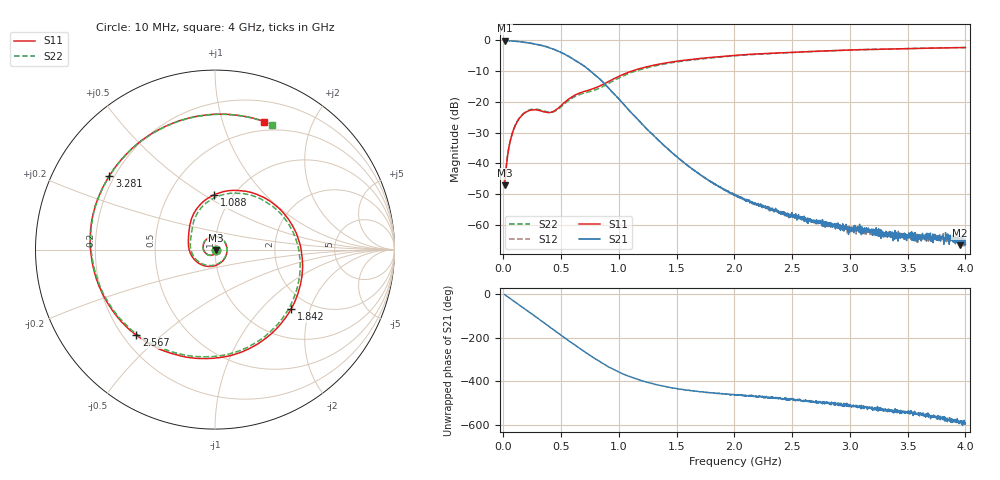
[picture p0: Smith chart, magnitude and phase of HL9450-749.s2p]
! 7/13/2020 7:49:31 AM
! H:\PRODUCTION_DATA\9450\10010\HL9450_10009_467MHZ_.S2P
! CHANNEL.1
! TR.MEASUREMENT
! CORRECTED.DATA
# GHZ S RI R 50.0
! FREQ.GHZ  S11RE  S11IM  S21RE  S21IM  S12RE  S12IM  S22RE  S22IM
!; PortSelection: Port_12
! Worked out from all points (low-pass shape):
!   2000 points, 10 MHz to 4 GHz, reference 50 ohm
!   highest |S21| = -0.04 dB at 10 MHz (marker M1); lowest = -66.7 dB at 3.952 GHz (marker M2)
!   |S21| within 3 dB of the highest: start of sweep to 444.1 MHz
!   lowest |S11| = -47.2 dB at 10 MHz (marker M3), VSWR 1.01, Z = 50.4 - j0.132 ohm
!   |S11| at or under -10 dB: start of sweep to 1.112 GHz
!   |S22| runs from -47.2 to -2.3 dB; largest |S21 - S12| = 0.0036
!   S11 on the Smith chart (normalised r, x): 10 MHz: 1.01, -0.00; 1.088 GHz: 0.82, +0.55; 1.842 GHz: 1.61, -1.50; 2.567 GHz: 0.25, -0.42; 3.281 GHz: 0.18, +0.31; 4 GHz: 0.40, +1.38
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0.01  0.00419 -0.00131  0.9926 -0.068  0.9946 -0.0685  0.00417 -0.00131
0.08185593  -0.0125 -0.0303  0.8355 -0.5062  0.8354 -0.5069  -0.013 -0.0306
0.2036118  -0.0655 0.0229  0.2095 -0.8929  0.2095 -0.8938  -0.0666 0.0239
0.2914357  -0.0112 0.0727  -0.2885 -0.807  -0.2886 -0.8069  -0.0115 0.0746
0.3932316  0.0654 0.0125  -0.6554 -0.3927  -0.656 -0.3929  0.0655 0.0145
0.5449275  -0.0449 -0.0933  -0.5125 0.261  -0.5121 0.2617  -0.0444 -0.0877
0.6766633  -0.1422 -0.00551  -0.1048 0.3926  -0.1036 0.3925  -0.1349 0.00216
0.8383392  -0.1436 0.1127  0.1531 0.1729  0.1519 0.1743  -0.1282 0.1105
1.087839  -0.00595 0.3047  0.0694 -0.021  0.0695 -0.021  3.89e-05 0.2904
1.341331  0.3045 0.2715  0.013 -0.0199  0.0129 -0.0199  0.3009 0.2543
1.586838  0.4792 0.00273  0.00165 -0.0093  0.00168 -0.0092  0.4683 -0.011
1.842326  0.4244 -0.3301  -0.000322 -0.00446  -0.000312 -0.00447  0.4056 -0.3377
2.005998  0.2798 -0.4969  -0.000543 -0.00294  -0.00067 -0.00291  0.2565 -0.499
2.27945  -0.0746 -0.6068  -0.00072 -0.0017  -0.000709 -0.00172  -0.0988 -0.5958
2.566873  -0.4378 -0.4779  -0.000777 -0.00103  -0.000826 -0.00109  -0.4573 -0.4546
2.670665  -0.5406 -0.3791  -0.000836 -0.000859  -0.000668 -0.00093  -0.5554 -0.3515
2.984037  -0.6952 0.0171  -0.000635 -0.000454  -0.000763 -0.000471  -0.6925 0.0533
3.281441  -0.588 0.4117  -0.000698 -0.000151  -0.000677 -0.000193  -0.565 0.4444
3.335333  -0.5466 0.4715  -0.000693 -4.72e-05  -0.000667 -4.84e-05  -0.52 0.5018
3.652696  -0.196 0.7185  -0.000547 0.000201  -0.000607 0.000138  -0.1535 0.73
3.952096  0.2106 0.7329  -0.000322 0.000333  -0.000348 0.000341  0.2555 0.7191
4  0.274 0.7131  -0.000281 0.000379  -0.000283 0.000371  0.3178 0.6965
